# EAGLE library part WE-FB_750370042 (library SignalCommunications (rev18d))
WE-FB Flyback Transformer suitable for LT3573/ LT3574/ LT3575/ LT3748 Characteristics easy design in solution less external components needed small board space low cost no optocoupler needed! long term reliability voltage control no aging same external parts for different output voltages easy design of custom power supply due to standard circuit and change of transformers and two components for feedback loop Isolation voltage up to 2.5 kV Applications Isolated power design Sensor interfaces Isolated telecom converters Power over Ethernet Details see: http://katalog.we-online.de/en/pbs/WE-FB_Linear? Updated 2014-07-07 2014 (C) Wurth Elektronik
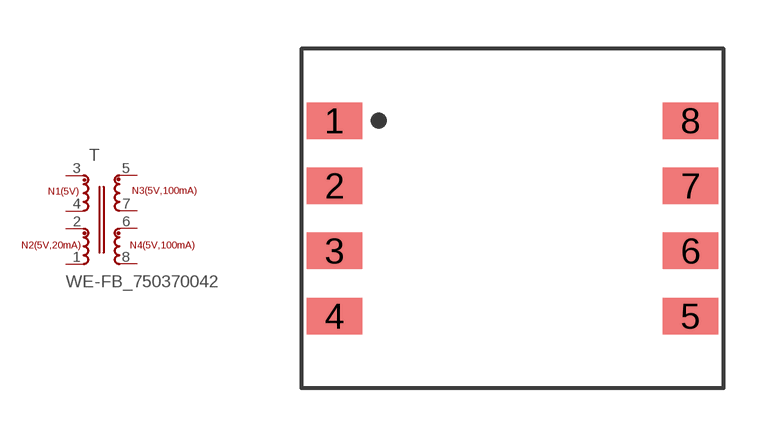
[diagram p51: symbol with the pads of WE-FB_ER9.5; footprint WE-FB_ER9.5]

Designator prefix T

## WE-FB_750370042  [WE-FB_ER9.5]
1  6  pas
2  7  pas
3  1  pas
4  8  pas
5  2  pas
6  4  pas
7  3  pas
8  5  pas

## Footprint WE-FB_ER9.5 (pad centres in mm)
smd 1.7 x 1.12: 1 -5.46,3; 2 -5.46,1; 3 -5.46,-1; 4 -5.46,-3; 5 5.46,-3; 6 5.46,-1; 7 5.46,1; 8 5.46,3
